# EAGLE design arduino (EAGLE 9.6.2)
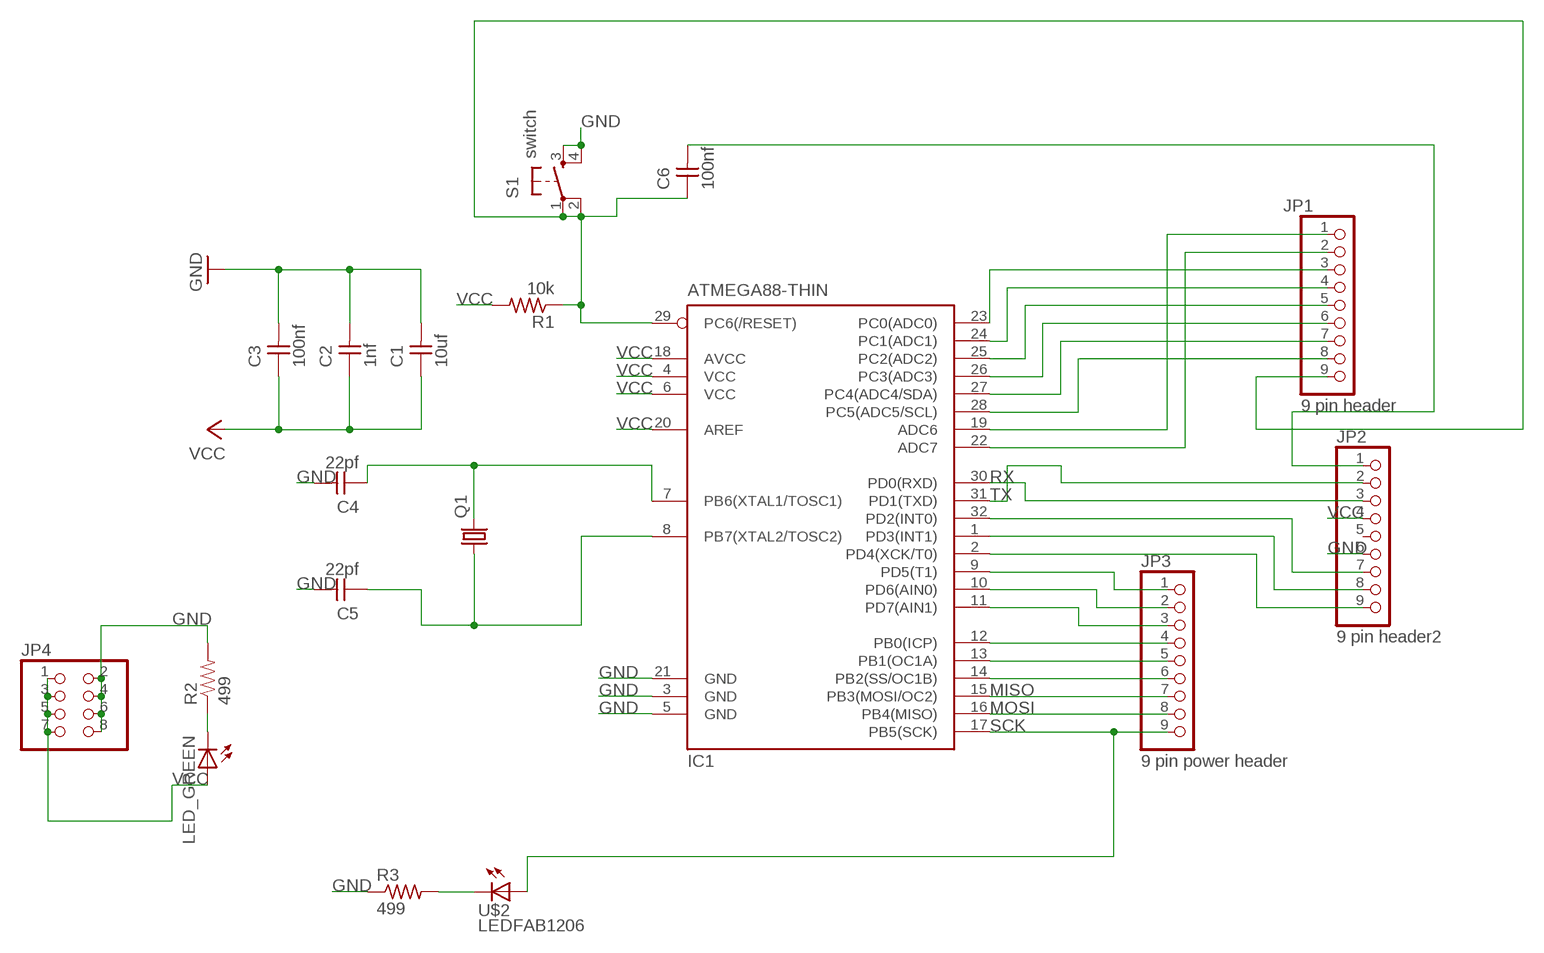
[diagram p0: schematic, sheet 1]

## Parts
C1  10uf  CAP-UNPOLARIZEDFAB  [C1206FAB]
C2  1nf  CAP-UNPOLARIZEDFAB  [C1206FAB]
C3  100nf  CAP-UNPOLARIZEDFAB  [C1206FAB]
C4  22pf  CAP-UNPOLARIZEDFAB  [C1206FAB]
C5  22pf  CAP-UNPOLARIZEDFAB  [C1206FAB]
C6  100nf  CAP-UNPOLARIZEDFAB  [C1206FAB]
IC1  ATMEGA88-THIN  [TQFP32-08THIN]
JP1  9 pin header  PINHD-1X9  [1X09]
JP2  9 pin header2  PINHD-1X9  [1X09]
JP3  9 pin power header  PINHD-1X9  [1X09]
JP4  PINHD-2X4  [2X04]
LED_GREEN  LED1206  [1206]
Q1  CRYSTALHC49S  [HC49/S]
R1  10k  RES-US1206FAB  [R1206FAB]
R2  499  RESISTOR1206  [1206]
R3  499  RES-US1206FAB  [R1206FAB]
S1  switch  6MM_SWITCH6MM_SWITCH  [6MM_SWITCH]
U$2  LEDFAB1206  [LED1206FAB]

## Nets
GND: C1.2 C2.2 C3.2 C4.2 C5.2 IC1.3(GND) IC1.5(GND) IC1.21(GND) JP2.6 JP4.2 JP4.4 JP4.6 JP4.8 R2.2 R3.1 S1.3(S) S1.4(S1)
MISO: IC1.15(PB3(MOSI/OC2)) JP3.7
MOSI: IC1.16(PB4(MISO)) JP3.8
N$1: IC1.23(PC0(ADC0)) JP1.3
N$2: IC1.24(PC1(ADC1)) JP1.4
N$3: IC1.25(PC2(ADC2)) JP1.5
N$4: IC1.26(PC3(ADC3)) JP1.6
N$5: IC1.27(PC4(ADC4/SDA)) JP1.7
N$6: IC1.28(PC5(ADC5/SCL)) JP1.8
N$7: C6.2 JP2.1
N$8: C6.1 IC1.29(PC6(/RESET)) JP1.9 R1.1 S1.1(P) S1.2(P1)
N$9: IC1.22(ADC7) JP1.2
N$10: IC1.19(ADC6) JP1.1
N$11: IC1.2(PD4(XCK/T0)) JP2.9
N$12: IC1.1(PD3(INT1)) JP2.8
N$13: IC1.32(PD2(INT0)) JP2.7
N$16: IC1.9(PD5(T1)) JP3.1
N$17: IC1.10(PD6(AIN0)) JP3.2
N$18: IC1.11(PD7(AIN1)) JP3.3
N$19: IC1.12(PB0(ICP)) JP3.4
N$20: IC1.13(PB1(OC1A)) JP3.5
N$21: IC1.14(PB2(SS/OC1B)) JP3.6
N$23: LED_GREEN.2(C) R2.1
N$26: R3.2 U$2.2(C)
N$30: C4.1 IC1.7(PB6(XTAL1/TOSC1)) Q1.2
N$31: C5.1 IC1.8(PB7(XTAL2/TOSC2)) Q1.1
RX: IC1.30(PD0(RXD)) JP2.3
SCK: IC1.17(PB5(SCK)) JP3.9 U$2.1(A)
TX: IC1.31(PD1(TXD)) JP2.2
VCC: C1.1 C2.1 C3.1 IC1.4(VCC) IC1.6(VCC) IC1.18(AVCC) IC1.20(AREF) JP2.4 JP4.1 JP4.3 JP4.5 JP4.7 LED_GREEN.1(A) R1.2
Unconnected: JP2.5

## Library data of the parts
C1-C6 = fab:CAP-UNPOLARIZED
IC1 = fab:ATMEGA88-THIN
JP1-JP3 = pinhead:PINHD-1X9: PIN HEADER
JP4 = pinhead:PINHD-2X4: PIN HEADER
LED_GREEN = 01_FAB_Hello:LED
Q1 = crystal:CRYSTAL: CRYSTAL; OC_FARNELL: 1667008; OC_NEWARK: unknown
R1 R3 = fab:RES-US: Resistor (US Symbol)
R2 = 01_SparkFun:RESISTOR: Resistor
S1 = fab:6MM_SWITCH: OMRON SWITCH
U$2 = fab:LED: LED

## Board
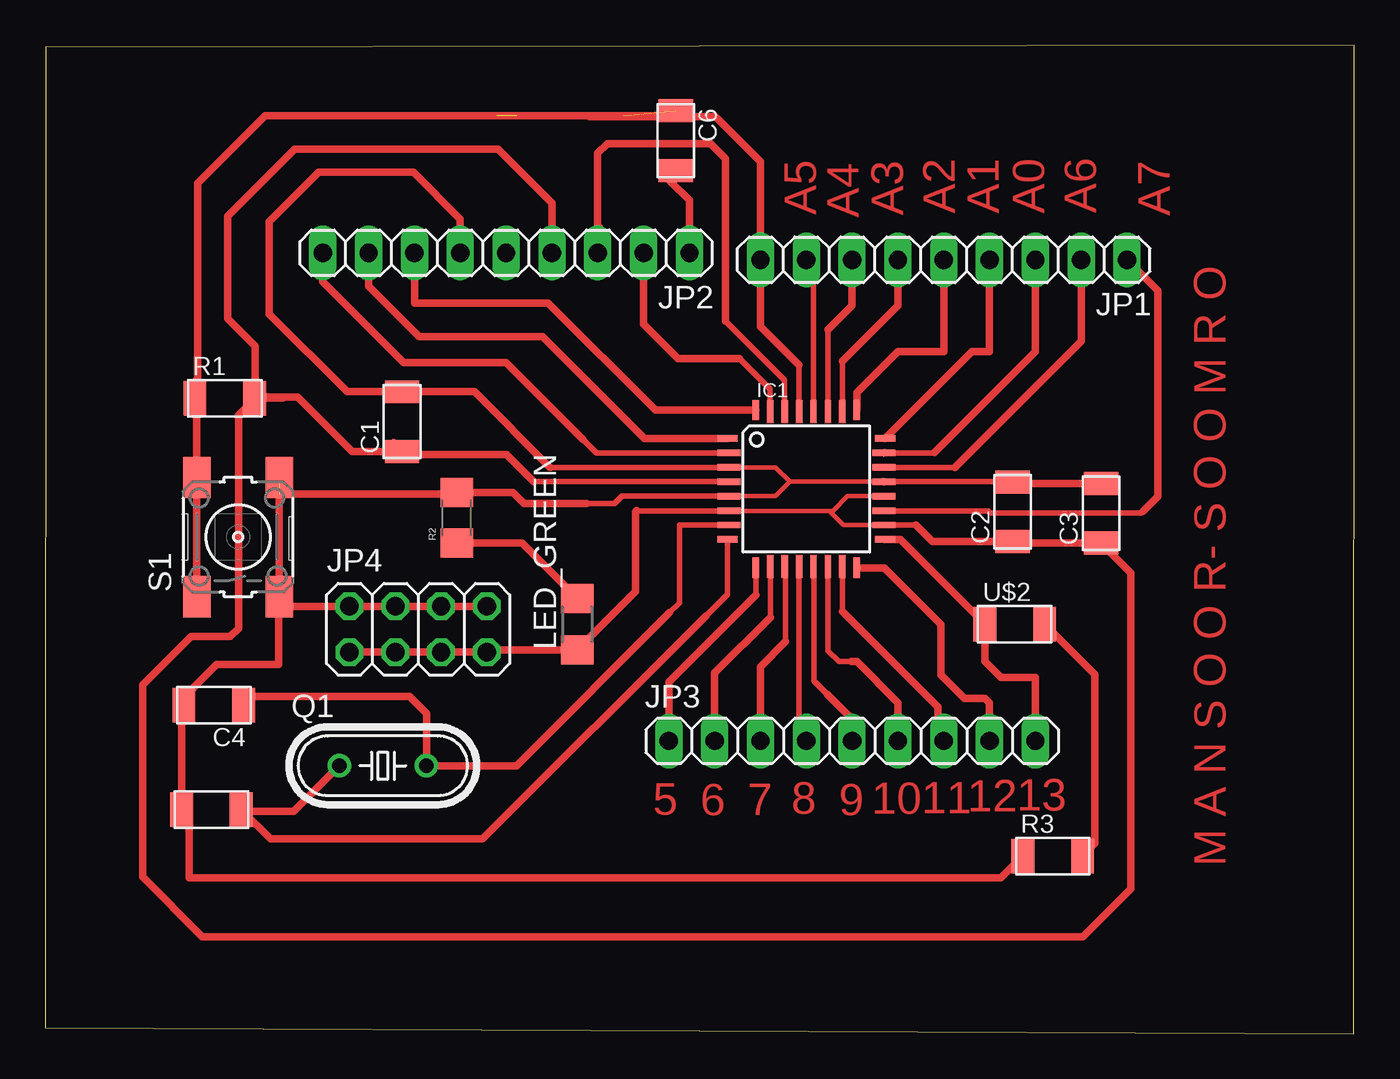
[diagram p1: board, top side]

Size 72.57 x 54.8 mm. Coordinates in mm from the lower left corner, seen from the top.
Outline: 0,0.33 72.54,0 72.57,54.8 0.03,54.68 0,0.33
Copper layers (1*16): Top 0.035mm / dielectric 1.5mm / Bottom 0.035mm
Design rules "default *": minimum track width 10mil, minimum drill 24mm, track to track 8mil, track to pad 8mil, pad to pad 8mil, via to via 8mil, smd to smd 8mil, copper to edge 40mil, drill to drill 8mil, minimum pad ring 10mil, minimum via ring 8mil, stop-mask expansion 4mil, vias tented up to drill 0mil, thermal gap 10mil

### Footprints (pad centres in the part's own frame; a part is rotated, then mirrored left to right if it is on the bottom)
C1206FAB = smd 1.27 x 1.905: 1 -1.651,0; 2 1.651,0
TQFP32-08THIN = smd 1.118 x 0.356: 1 -4.369,2.8; 8 -4.369,-2.8; 17 4.369,-2.8; 24 4.369,2.8 | smd 1.27 x 0.356: 2 -4.293,2; 3 -4.293,1.2; 4 -4.293,0.4; 5 -4.293,-0.4; 6 -4.293,-1.2; 7 -4.293,-2; 18 4.293,-2; 19 4.293,-1.2; 20 4.293,-0.4; 21 4.293,0.4; 22 4.293,1.2; 23 4.293,2 | smd 0.356 x 1.118: 9 -2.8,-4.369; 16 2.8,-4.369; 25 2.8,4.369; 32 -2.8,4.369 | smd 0.356 x 1.27: 10 -2,-4.293; 14 1.2,-4.293; 15 2,-4.293; 26 2,4.293; 27 1.2,4.293; 31 -2,4.293 | smd 0.35 x 1.27: 11 -1.2,-4.293; 12 -0.4,-4.293; 13 0.4,-4.293; 28 0.4,4.293; 29 -0.4,4.293; 30 -1.2,4.293
1X09 = drill 1.016 long: 1 -10.16,0; 2 -7.62,0; 3 -5.08,0; 4 -2.54,0; 5 0,0; 6 2.54,0; 7 5.08,0; 8 7.62,0; 9 10.16,0
2X04 = drill 1.016 octagon: 1 -3.81,-1.27; 2 -3.81,1.27; 3 -1.27,-1.27; 4 -1.27,1.27; 5 1.27,-1.27; 6 1.27,1.27; 7 3.81,-1.27; 8 3.81,1.27
1206 = smd 1.6 x 1.803: 1 -1.422,0; 2 1.422,0
HC49/S = drill 0.813: 1 -2.413,0; 2 2.413,0
R1206FAB = smd 1.27 x 1.905: 1 -1.651,0; 2 1.651,0
1206' = smd 1.6 x 1.8: 1 -1.4,0; 2 1.4,0
6MM_SWITCH = smd 2.286 x 1.524: 1 -3.302,2.286; 2 3.302,2.286; 3 -3.302,-2.286; 4 3.302,-2.286
LED1206FAB = smd 1.27 x 1.905: 1 -1.651,0; 2 1.651,0

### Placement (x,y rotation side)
C1  19.79,33.93 90 top
C2  53.62,28.93 90 top
C3  58.52,28.85 90 top
C4  9.35,18.21 180 top
C5  9.22,12.42 180 top
C6  34.95,49.5 270 top
IC1  42.19,30.2 0 top
JP1  49.81,42.9 180 top
JP2  25.55,43.28 180 top
JP3  44.73,16.23 0 top
JP4  20.68,22.43 0 top
LED_GREEN  29.49,22.71 90 top
Q1  18.72,14.86 0 top
R1  9.96,35.23 0 top
R2  499  [1206']  22.81,28.6 90 top
R3  55.85,9.86 0 top
S1  10.69,27.53 90 top
U$2  53.75,22.71 0 top

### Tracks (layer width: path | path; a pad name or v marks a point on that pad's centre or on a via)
GND  (1 unrouted)
  Top 0.254: IC1.21 41.28,30.6 | IC1.3 40.48,31.4 41.28,30.6 | 41.28,30.6 40.48,29.8 IC1.5
  Top 0.305: 27.98,31.4 IC1.3 | 30,29.39 31.57,29.39 31.99,29.8 IC1.5 | IC1.21 53.6,30.6 C2.2
  Top 0.406: 46.5,30.58 IC1.21 | C3.2 53.7,30.51 C2.2 | R3.1 52.98,8.64 7.98,8.64 7.98,12.01 C5.2 7.57,18.08 C4.2 7.7,18.67 9.5,20.47 12.95,20.47 12.95,24.21 S1.3 | 27.98,31.4 23.8,35.59 C1.2 16.74,35.59 12.42,39.9 12.42,45.01 15.16,47.75 20.42,47.75 23.01,45.16 JP2.6 | R2.2 23.01,29.8 | S1.3 12.98,24.41 13.69,23.7 JP4.2 JP4.4 JP4.6 JP4.8 | 12.98,30.63 13.21,30.86 13,30.86 S1.4 S1.3 | R2.2 22.73,29.92 12.98,29.92 | R2.2 25.93,30 26.54,29.39 30,29.39
MISO
  Top 0.305: 44.19,23.4 IC1.15
  Top 0.406: JP3.7 49.48,16.56 49.48,18.11 44.19,23.4
MOSI
  Top 0.406: IC1.16 46.51,25.83 49.66,22.68 49.66,19.89 50.95,18.59 52.1,18.59 52.35,18.34 JP3.8
N$1
  Top 0.305: 49.29,32.23 49.27,32.2 IC1.23
  Top 0.406: IC1.23 46.51,32.23 | 49.29,32.23 54.89,37.82 JP1.3
N$2
  Top 0.406: IC1.24 51.38,37.82 52.35,37.82 JP1.4
N$3
  Top 0.406: IC1.25 44.99,35.54 47.27,37.82 49.81,37.82 JP1.5
N$4
  Top 0.305: 44.19,37.28 IC1.26
  Top 0.406: 44.19,37.28 47.27,40.36 JP1.6
N$5
  Top 0.305: 43.39,39.02 IC1.27
  Top 0.406: 43.39,39.02 44.73,40.36 JP1.7
N$6
  Top 0.305: IC1.28 42.59,42.5
  Top 0.406: 42.59,42.5 JP1.8
N$7
  Top 0.406: C6.2 34.65,47.27 35.71,46.2 JP2.1
N$8  (2 unrouted)
  Top 0.254: 32.05,50.88 32.11,50.83
  Top 0.305: 41.79,37.08 IC1.29
  Top 0.406: S1.1 S1.2 8.41,35.23 | 8.41,36.27 8.41,35.97 | 8.41,35.97 8.41,35.23 | 26.16,50.88 12.19,50.88 8.46,47.14 8.46,36.02 8.41,35.97 | 41.79,37.08 39.66,39.21 39.66,41.65 39.65,41.66 JP1.9 39.65,48.34 37.16,50.83 34.16,50.83 | 30.18,50.83 30.48,50.83 | 31.01,50.83 32.11,50.83 34.16,50.83 | 8.41,35.23 R1.1 | 25.02,50.88 28.8,50.88 30.43,50.88 | 30.43,50.88 30.96,50.88 31.01,50.83 | 31.01,50.83 30.48,50.83 | 30.48,50.83 30.43,50.88 | 30.43,50.88 34.11,50.88 34.16,50.83
N$9
  Top 0.305: 50.43,31.4 IC1.22
  Top 0.406: JP1.2 57.43,38.4 50.43,31.4
N$10
  Top 0.305: IC1.19 46.63,29 46.66,28.98 52.28,28.98 52.37,28.88 60.76,28.88 60.86,28.98
  Top 0.406: JP1.1 61.67,41.2 61.67,29.79 60.86,28.98
N$11
  Top 0.305: 29.82,32.94 30.56,32.2 IC1.2
  Top 0.406: JP2.9 15.39,41.68 19.86,37.21 25.55,37.21 29.82,32.94
N$12
  Top 0.406: IC1.1 33.22,33 27.56,38.66 20.73,38.66 17.93,41.45 JP2.8
N$13
  Top 0.406: IC1.32 33.83,34.57 27.89,40.51 20.47,40.51 JP2.7
N$16
  Top 0.305: 39.4,24.33 IC1.9
  Top 0.406: JP3.1 34.57,19.51 39.4,24.33
N$17
  Top 0.305: 40.21,23.09 40.21,25.89 IC1.10
  Top 0.406: JP3.2 37.11,19.99 40.21,23.09
N$18
  Top 0.305: 41.05,21.74 41.05,25.85 IC1.11
  Top 0.406: JP3.3 39.65,20.35 41.05,21.74
N$19
  Top 0.305: JP3.4 41.79,16.63 IC1.12
  Top 0.406: JP3.4 41.78,16.64
N$20
  Top 0.305: 43.36,18.82 42.62,19.56 42.62,25.88 IC1.13
  Top 0.406: JP3.5 44.73,17.45 43.36,18.82
N$21
  Top 0.305: IC1.14 43.39,21.23 43.99,20.62 44.68,20.62
  Top 0.406: JP3.6 47.27,18.34 44.98,20.62 44.68,20.62
N$23
  Top 0.406: 29.87,24.51 LED_GREEN.2 29.49,24.15 26.44,27.2 R2.1
N$26
  Top 0.406: R3.2 58.19,10.54 58.19,19.91 U$2.2
N$30
  Top 0.305: 34.62,23.34 35.15,23.88 35.15,28.19 35.16,28.2 IC1.7
  Top 0.406: C4.1 11.48,18.69 20.19,18.69 21.13,17.75 Q1.2 26.14,14.86 34.62,23.34
N$31
  Top 0.305: 36.63,23.16 37.82,24.36 IC1.8
  Top 0.406: IC1.8 | 10.96,12.33 12.5,10.79 24.26,10.79 36.63,23.16 | 10.96,12.33 C5.1 | Q1.1 13.78,12.33 10.96,12.33
RX
  Top 0.305: IC1.30 40.99,36.23 37.72,39.5 | 30.78,44.7 30.63,44.55 JP2.3
  Top 0.406: JP2.3 30.63,48.82 31.17,49.35 36.88,49.35 37.72,48.51 37.72,39.5
SCK
  Top 0.406: IC1.17 47.4,27.4 U$2.1 52.1,20.65 52.98,19.76 54.89,19.76 JP3.9
TX
  Top 0.305: IC1.31 40.19,35.73 38.48,37.44
  Top 0.406: 38.48,37.44 35.08,37.44 33.17,39.34 JP2.2
VCC
  Top 0.254: IC1.20 44.48,29.8 43.66,28.98 43.46,28.98 | IC1.6 37.92,28.98 43.46,28.98 | IC1.18 44.24,28.2 43.46,28.98
  Top 0.305: 32.72,28.93 32.77,28.98 37.92,28.98 | 27.08,30.6 IC1.4 | 48.25,28.2 IC1.18
  Top 0.406: C2.1 53.29,27.28 | 53.29,27.28 49.17,27.28 48.25,28.2 | C3.1 53.37,27.2 53.29,27.28 | 32.79,29 32.72,28.93 32.72,24.51 LED_GREEN.1 24.61,21.29 JP4.7 JP4.5 JP4.3 JP4.1 | C1.1 19.3,32.77 | C1.1 19.96,32.11 25.58,32.11 27.08,30.6 | C1.1 19.79,32.56 | C3.1 58.98,27.2 | C1.1 17.02,32.28 14,35.31 13.18,35.31 | JP2.4 28.09,46.05 25.1,49.05 13.84,49.05 10.11,45.31 10.11,39.63 11.63,38.11 11.63,35.31 13.18,35.31 | 11.66,35.23 13.18,35.23 13.18,35.31 | 11.66,35.23 R1.2 | 11.66,35.23 10.72,34.29 10.72,22.48 10.26,22.02 8.1,22.02 5.41,19.33 5.41,8.69 8.71,5.38 57.53,5.38 60.17,8.03 60.17,25.55 C3.1

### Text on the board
Top: A5 | A4 | A3 | A2 | A1 | A0 | A6 | A7 | 5 | 6 | 7 | 8 | 9 | 10 | 11 | 12 | 13 | M A N S O O R- S O O M R O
